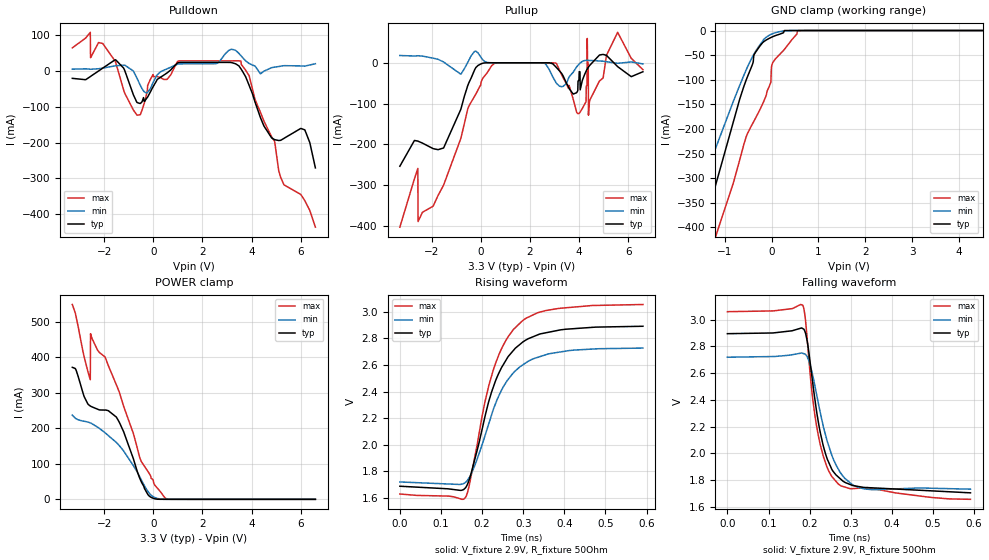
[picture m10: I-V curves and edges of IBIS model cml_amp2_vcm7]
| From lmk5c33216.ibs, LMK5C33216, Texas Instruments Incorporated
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[Model]   cml_amp2_vcm7
Model_type   Output
Polarity   Non-Inverting
Vmeas = 2.25
Vref = 2.9
Cref = 0pF
Rref = 50
|   typ   min   max
C_comp   0.65pF   0.575pF   0.725pF
[Voltage Range]   3.3   3.135   3.465
[Temperature Range]   50   135   -40
[Pullup Reference]   3.3   3.135   3.465
[Pulldown Reference]   0   0   -0
[Power Clamp Reference]   3.3   3.135   3.465
[GND Clamp Reference]   0   0   0
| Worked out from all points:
|   slope of the pulldown table from 0 to 0.495 V, typ, clamps not added: 14.3 ohm
|   falling waveform, V_fixture 2.9V, R_fixture 50Ohm: 20-80 % time 42.8ps typ, 50ps min, 41.6ps max; typ from 2.9 V to 1.7 V
|   rising waveform, V_fixture 2.9V, R_fixture 50Ohm: 20-80 % time 75.4ps typ, 80.7ps min, 72.6ps max; typ from 1.69 V to 2.89 V
[Pulldown]
|   Voltage   I(typ)   I(min)   I(max)
-3.3V     -20.59mA   5.077mA    64.69mA
-2.567V   -15.76mA   4.918mA    108.1mA
-2.062V   7.911mA    8.065mA    77.04mA
-1.528V   30.76mA    14.66mA    22.55mA
-656.7mV  -88.38mA   -21.44mA   -123.5mA
-13.2mV   -44.48mA   -32.67mA   -9.952mA
986.7mV   22.44mA    18.83mA    26.85mA
3.571V    5.802mA    42.7mA     27.85mA
4.818V    -187.2mA   9.247mA    -184mA
5.313V    -188.8mA   14.8mA     -317.1mA
6.164V    -164.5mA   13.59mA    -361.8mA
6.6V      -270.9mA   20.32mA    -436.6mA
[GND Clamp]
|   Voltage   I(typ)   I(min)   I(max)
-3.3V     -1.161A    -986.5mA   -1.48A
-1.795V   -504mA     -421.6mA   -669.2mA
-1.508V   -420.3mA   -321mA     -551.3mA
-1.409V   -387.6mA   -293.5mA   -510.5mA
-1.211V   -320.6mA   -244.1mA   -424.5mA
-815.1mV  -186.1mA   -144.2mA   -310.3mA
-537.9mV  -99.97mA   -79.46mA   -215.4mA
-369.6mV  -48.73mA   -47.08mA   -183.3mA
-23.1mV   -14.69mA   -8.348mA   -107.4mA
6.6mV     -13.36mA   -7.036mA   -70.49mA
570.9mV   0A         -9.437uA   -391.2uA
6.6V      0A         0A         0A
[Pullup]
|   Voltage   I(typ)   I(min)   I(max)
-3.3V     -254.1mA   17.84mA    -403.7mA
-2.567V   -192.3mA   17.27mA    -259.5mA
-2.558V   -192.6mA   17.26mA    -389.9mA
-1.944V   -210.8mA   11.4mA     -352.2mA
570.9mV   -565.7nA   10.81uA    -391.3uA
3.056V    -10.16mA   -48.29mA   -873.2uA
3.977V    -43.7mA    -4.692mA   -124.7mA
4.283V    -21mA      5.89mA     -95.59mA
4.333V    -15.27mA   5.761mA    59.66mA
4.382V    -10.55mA   5.651mA    -128.7mA
5.57V     -9.446mA   -1.233mA   74.82mA
6.6V      -21.95mA   -2.704mA   -16.95mA
[POWER Clamp]
|   Voltage   I(typ)   I(min)   I(max)
-3.3V     371.7mA    237.1mA    548.6mA
-3.151V   364.5mA    227.2mA    516.2mA
-2.815V   288.8mA    219.8mA    400.7mA
-2.567V   262.8mA    215.2mA    336.7mA
-2.558V   262.4mA    214.9mA    466.5mA
-2.27V    253.8mA    203.2mA    420mA
-1.964V   251.4mA    187.3mA    399.9mA
-1.508V   231.7mA    160.3mA    322.9mA
-537.9mV  56.76mA    61.47mA    114.3mA
-221.1mV  13.55mA    22.33mA    78.67mA
481.8mV   75.9uA     118.2uA    3.912mA
6.6V      0A         0A         0A
[Ramp]
R_load = 50
|   typ   min   max
dV/dt_r   0.721182/7.50792e-11   0.603535/8.03923e-11   0.854329/7.25273e-11
dV/dt_f   0.715725/4.23893e-11   0.593298/4.98886e-11   0.84382/4.13687e-11
[Falling Waveform]
V_fixture = 2.9V
V_fixture_min = 2.735V
V_fixture_max = 3.065V
R_fixture = 50Ohm
C_fixture = 0F
|   Time   V(typ)   V(min)   V(max)
0s        2.896V     2.719V     3.061V
182.9ps   2.935V     2.749V     3.111V
188.3ps   2.915V     2.744V     3.041V
194ps     2.843V     2.723V     2.861V
207.6ps   2.525V     2.581V     2.405V
221.3ps   2.232V     2.373V     2.13V
242.9ps   1.956V     2.089V     1.892V
269.8ps   1.822V     1.881V     1.769V
332.5ps   1.744V     1.733V     1.74V
591.2ps   1.703V     1.731V     1.655V
[Rising Waveform]
V_fixture = 2.9V
V_fixture_min = 2.735V
V_fixture_max = 3.065V
R_fixture = 50Ohm
C_fixture = 0F
|   Time   V(typ)   V(min)   V(max)
0s        1.689V     1.721V     1.63V
158.9ps   1.675V     1.716V     1.601V
168.4ps   1.735V     1.751V     1.689V
182.5ps   1.893V     1.847V     1.912V
206.1ps   2.2V       2.059V     2.31V
226.7ps   2.428V     2.26V      2.556V
257.9ps   2.635V     2.467V     2.784V
298.2ps   2.77V      2.599V     2.932V
409.7ps   2.87V      2.707V     3.031V
591.2ps   2.891V     2.727V     3.054V
